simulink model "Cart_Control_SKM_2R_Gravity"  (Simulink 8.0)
settings: Solver=FixedStepDiscrete  SolverMode=SingleTasking  StartTime=0  StopTime=6  FixedStep=dt  RelTol=1e-3  SampleTimeConstraint=Specified
InitFcn:
  | % Sampling Times %
  | dt0=0.001; dt1=0.01; samples=10;
undefined symbols (not defined in the file or in its folder): DiscIntNeverNeededParam, Volts
libraries: simulink_extras x4, speedgoatlib_IO311 x3, speedgoatlib_IO101 x2, simulink x2, xpclib x1

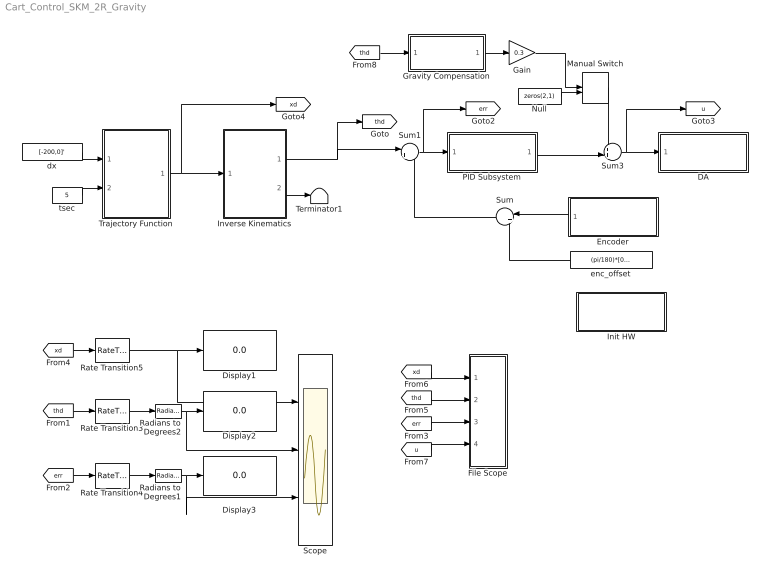
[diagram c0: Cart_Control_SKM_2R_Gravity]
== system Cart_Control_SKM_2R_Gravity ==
  DA : Subsystem  TreatAsAtomicUnit=on
  Display1 : Display
  Display2 : Display
  Display3 : Display
  Encoder : Subsystem  TreatAsAtomicUnit=on
  File Scope : Subsystem
  Gain : Gain  Gain=0.3
  Gravity Compensation : MATLAB Function  TreatAsAtomicUnit=on
  Init HW : Subsystem  TreatAsAtomicUnit=on
  Inverse Kinematics : MATLAB Function  TreatAsAtomicUnit=on
  Manual Switch : ManualSwitch
  Null : Constant  Value=zeros(2,1)
  PID Subsystem : Subsystem  TreatAsAtomicUnit=on
  Radians to Degrees1 : simulink_extras/Transformations/Radians to Degrees
  Radians to Degrees2 : simulink_extras/Transformations/Radians to Degrees
  Rate Transition3 : RateTransition  OutPortSampleTime=dt1
  Rate Transition4 : RateTransition  OutPortSampleTime=dt1
  Rate Transition5 : RateTransition  OutPortSampleTime=dt1
  Scope : Scope  NumInputPorts=3
  Sum : Sum  Inputs=|++
  Sum1 : Sum  Inputs=|+-
  Sum3 : Sum  Inputs=++|
  Terminator1 : Terminator
  Trajectory Function : MATLAB Function  TreatAsAtomicUnit=on
  dx : Constant  Value=[-200,0]'  SampleTime=dt0
  enc_offset : Constant  Value=(pi/180)*[0,90]'
  tsec : Constant  Value=5  SampleTime=dt0
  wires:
  Sum1/1 -> PID Subsystem/1(In1), [err]
  PID Subsystem/1(Out1) -> Sum3/2
  Encoder/1(Out1) -> Sum/1
  enc_offset/1 -> Sum/2
  Sum/1 -> Sum1/2
  [xd] -> File Scope/1(xd)
  [thd] -> File Scope/2(thd)
  [err] -> File Scope/3(err)
  [u] -> File Scope/4(u)
  dx/1 -> Trajectory Function/1(dx)
  tsec/1 -> Trajectory Function/2(tsec)
  Trajectory Function/1(xd) -> [xd], Inverse Kinematics/1(xd)
  Inverse Kinematics/1(thd) -> Sum1/1, [thd]
  [thd] -> Rate Transition3/1
  [err] -> Rate Transition4/1
  [xd] -> Rate Transition5/1
  Rate Transition5/1 -> Display1/1, Scope/1
  Rate Transition3/1 -> Radians to Degrees2/1
  Rate Transition4/1 -> Radians to Degrees1/1
  Radians to Degrees2/1 -> Display2/1, Scope/2
  Radians to Degrees1/1 -> Display3/1, Scope/3
  Inverse Kinematics/2(w_index) -> Terminator1/1
  Sum3/1 -> DA/1(In1), [u]
  Manual Switch/1 -> Sum3/1
  Null/1 -> Manual Switch/2
  [thd] -> Gravity Compensation/1(thd)
  Gravity Compensation/1(out) -> Gain/1
  Gain/1 -> Manual Switch/1

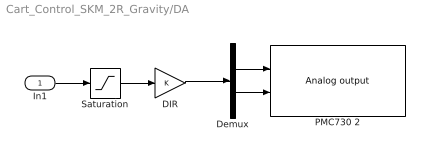
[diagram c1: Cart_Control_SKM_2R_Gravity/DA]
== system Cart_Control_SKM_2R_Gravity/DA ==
  In1 : Inport
  DIR : Gain
  Demux : Demux  Outputs=2
  PMC730 2 : speedgoatlib_IO101/Analog output  id=1  channel=[1,2]  reset=[1,1]  initValue=[0,0]  ts=dt0  pciSlot=-1
  Saturation : Saturate  UpperLimit=10  LowerLimit=-10
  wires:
  In1/1 -> Saturation/1
  Saturation/1 -> DIR/1
  DIR/1 -> Demux/1
  Demux/2 -> PMC730 2/2
  Demux/1 -> PMC730 2/1

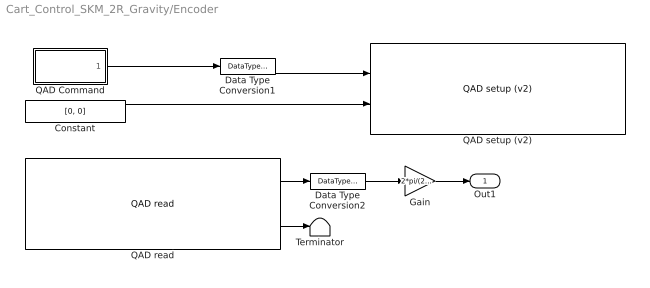
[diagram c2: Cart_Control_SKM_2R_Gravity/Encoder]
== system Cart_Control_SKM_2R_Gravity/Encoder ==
  Constant : Constant  Value=[0, 0]  OutDataTypeStr=Inherit: Inherit via back propagation
  Data Type Conversion1 : DataTypeConversion  OutDataTypeStr=uint8
  Data Type Conversion2 : DataTypeConversion  OutDataTypeStr=double
  Gain : Gain  Gain=2*pi/(23*2000)
  QAD Command : MATLAB Function  TreatAsAtomicUnit=on
  QAD read : speedgoatlib_IO311/QAD/QAD read  id=1  chan=[1 2]  pciSlot=-1  ts=dt0
  QAD setup (v2) : speedgoatlib_IO311/QAD/QAD setup (v2)  id=1  chan=[1,2]  debounce=0  quadrature=4x  index=Ignore index input  special=Disabled (cycling counter)  steps=2000  ts=dt0  pciSlot=-1
  Terminator : Terminator
  Out1 : Outport
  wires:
  Gain/1 -> Out1/1
  Constant/1 -> QAD setup (v2)/2
  QAD read/2 -> Terminator/1
  QAD read/1 -> Data Type Conversion2/1
  QAD Command/1(y) -> Data Type Conversion1/1
  Data Type Conversion2/1 -> Gain/1
  Data Type Conversion1/1 -> QAD setup (v2)/1

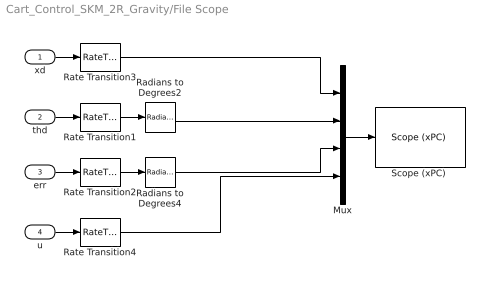
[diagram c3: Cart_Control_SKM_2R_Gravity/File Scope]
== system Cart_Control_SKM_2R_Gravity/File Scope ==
  xd : Inport
  thd : Inport  Port=2
  err : Inport  Port=3
  u : Inport  Port=4
  Mux : Mux
  Radians to Degrees2 : simulink_extras/Transformations/Radians to Degrees
  Radians to Degrees4 : simulink_extras/Transformations/Radians to Degrees
  Rate Transition{1..4} (4 alike) : RateTransition  OutPortSampleTime=dt1
  "Scope (xPC) " : xpclib/Misc./Scope (xPC)   scopeno=1  scopetype=File  autostart=on  viewmode=Graphical redraw  formatstr='%15.6f'  grid=on  ylimits=[0,0]  nosamples=100  noprepostsamples=0  interleave=1  triggermode=FreeRun  triggersignal=1  triggerlevel=0.0  triggerslope=Either  triggerscope=1  triggersample=0  filename=step2.dat  mode=Lazy  writesize=512  autorestart=on  dynamicfilemode=off  maxwritefilesize=512*1024^2
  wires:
  Radians to Degrees2/1 -> Mux/2
  Radians to Degrees4/1 -> Mux/3
  Rate Transition1/1 -> Radians to Degrees2/1
  Rate Transition2/1 -> Radians to Degrees4/1
  thd/1 -> Rate Transition1/1
  err/1 -> Rate Transition2/1
  Rate Transition3/1 -> Mux/1
  xd/1 -> Rate Transition3/1
  u/1 -> Rate Transition4/1
  Mux/1 -> "Scope (xPC) "/1
  Rate Transition4/1 -> Mux/4

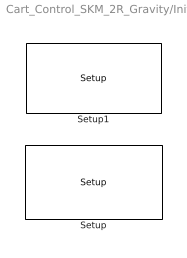
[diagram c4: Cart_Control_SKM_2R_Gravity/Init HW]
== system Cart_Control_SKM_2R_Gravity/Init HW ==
  Setup : speedgoatlib_IO311/Setup/Setup  group=Module setup  id=1  fpga1=speedgoat_IO311_default  pciSlot=-1  lowerDirection=[1 1 1 1 1 0 0 0 0 0 0 0 1 0 0 0]  lowerReset=[1]  lowerValue=[0]  upperDirection=[1 1 1 1 1 1 1 1 1 0 0 0 0 0 0 0]  upperReset=[1]  upperValue=[0]
  Setup1 : speedgoatlib_IO101/Setup  group=Module setup  id=1  pciSlot=-1  adStartChannel=1  adNumChannel=32  adCoupling=Single-ended  adRange=-10 .. 10 Volts  adAcqMode=Standard  daChannel=[1,2]  daReset=[1,1]  daInitValue=[0,0]  lowerChannel=1  lowerDirection=Input  lowerDIDebounce=0  lowerDOReset=[1]  lowerDOInitValues=[0]  upperChannel=1  upperDirection=Output  upperDIDebounce=0  upperDOReset=0  upperDOInitValues=0

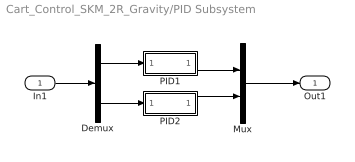
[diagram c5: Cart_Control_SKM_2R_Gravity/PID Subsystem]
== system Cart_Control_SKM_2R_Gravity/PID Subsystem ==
  In1 : Inport
  Demux : Demux  Outputs=2
  Mux : Mux  Inputs=2
  PID1 : Subsystem
  PID2 : Subsystem
  Out1 : Outport
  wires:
  In1/1 -> Demux/1
  Demux/1 -> PID1/1(In1)
  PID1/1(Out1) -> Mux/1
  Demux/2 -> PID2/1(In1)
  PID2/1(Out1) -> Mux/2
  Mux/1 -> Out1/1

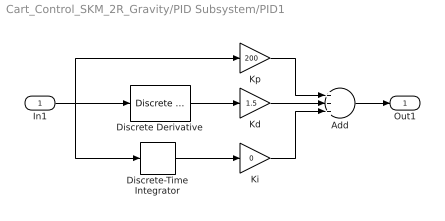
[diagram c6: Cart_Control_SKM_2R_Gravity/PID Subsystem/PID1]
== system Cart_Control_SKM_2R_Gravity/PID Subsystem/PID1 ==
  In1 : Inport
  Add : Sum  Inputs=+++
  Discrete Derivative : simulink/Discrete/Discrete Derivative  gainval=1.0  ICPrevScaledInput=0.0  InputProcessing=Inherited  OutMin=[]  OutMax=[]  OutDataType=fixdt(1, 16)  OutScaling=2^-10  DoSatur=off
  Discrete-Time Integrator : DiscreteIntegrator  SampleTime=dt0  ICPrevOutput=DiscIntNeverNeededParam  ICPrevScaledInput=DiscIntNeverNeededParam
  Kd : Gain  Gain=1.5
  Ki : Gain  Gain=0
  Kp : Gain  Gain=200
  Out1 : Outport
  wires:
  Discrete-Time Integrator/1 -> Ki/1
  Kp/1 -> Add/1
  Kd/1 -> Add/2
  Ki/1 -> Add/3
  Discrete Derivative/1 -> Kd/1
  Add/1 -> Out1/1
  In1/1 -> Kp/1, Discrete Derivative/1, Discrete-Time Integrator/1

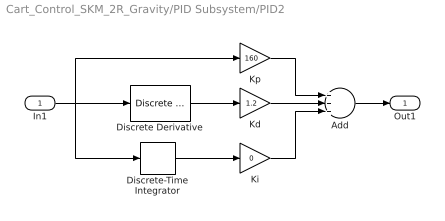
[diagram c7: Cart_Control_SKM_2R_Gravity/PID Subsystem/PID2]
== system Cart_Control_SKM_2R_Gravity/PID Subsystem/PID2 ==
  In1 : Inport
  Add : Sum  Inputs=+++
  Discrete Derivative : simulink/Discrete/Discrete Derivative  gainval=1.0  ICPrevScaledInput=0.0  InputProcessing=Inherited  OutMin=[]  OutMax=[]  OutDataType=fixdt(1, 16)  OutScaling=2^-10  DoSatur=off
  Discrete-Time Integrator : DiscreteIntegrator  SampleTime=dt0  ICPrevOutput=DiscIntNeverNeededParam  ICPrevScaledInput=DiscIntNeverNeededParam
  Kd : Gain  Gain=1.2
  Ki : Gain  Gain=0
  Kp : Gain  Gain=160
  Out1 : Outport
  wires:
  Discrete-Time Integrator/1 -> Ki/1
  Kp/1 -> Add/1
  Kd/1 -> Add/2
  Ki/1 -> Add/3
  Discrete Derivative/1 -> Kd/1
  Add/1 -> Out1/1
  In1/1 -> Kp/1, Discrete Derivative/1, Discrete-Time Integrator/1

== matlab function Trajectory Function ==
function xd = fcn(dx, tsec)

persistent index xd_p

MAX_CH=2;       % Two Actuators %
dt=0.001;       % Step time is 10 msec %
a1=100; a2=100;

% Initializing Variables %
if isempty(index), index=0; end
if isempty(xd_p), xd_p=zeros(MAX_CH,1); end
xd=zeros(MAX_CH,1);
x0=[a1,a2]';

tout=index*dt;
if index<(tsec/dt)
    [c] = coeff_3rd(x0, zeros(MAX_CH,1), x0+dx, zeros(MAX_CH,1), tsec);
    for ch=1:MAX_CH
        xd(ch,1)=c(ch,1)+c(ch,2)*tout+c(ch,3)*tout^2+c(ch,4)*tout^3;    
    end
    xd_p=xd;
else
    xd=xd_p;
end
index=index+1;

function [c] = coeff_3rd(sp, sv, ep, ev, tsec)
MAX_CH=2;
c=zeros(MAX_CH,4);
for ch=1:MAX_CH
    c(ch,1)=sp(ch,1);
    c(ch,2)=sv(ch,1);
    c(ch,3)=(3.0*(ep(ch,1)-sp(ch,1))-(2.0*sv(ch,1)+ev(ch,1))*tsec)/(tsec*tsec);
    c(ch,4)=(-2.0*(ep(ch,1)-sp(ch,1))+(sv(ch,1)+ev(ch,1))*tsec)/(tsec*tsec*tsec);
end

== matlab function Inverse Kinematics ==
function [thd,w_index]  = fcn(xd)

persistent index thd_p

% Initializing Variables %
if isempty(index), index=0; end
if isempty(thd_p), thd_p=(pi/180)*[0,90]'; end

w_index=1;  % In workspace %
a1=100; a2=100;

% (1) Calculate th2 %
px=xd(1,1); py=xd(2,1);
kapha=(px^2+py^2-a1^2-a2^2)/(2*a1*a2);
if abs(kapha)>1
    w_index=-1;  % Out of Workspace %
    kapha=1;
end
th2=+acos(kapha); % Elbow Down %
%th2=-acos(kapha); % Elbow Up %
 
% (2) Calculate th1 %
delta=a1^2+a2^2+2*a1*a2*cos(th2);
cth1=(px*(a1+a2*cos(th2))+py*a2*sin(th2))/delta;
sth1=(-px*a2*sin(th2)+py*(a1+a2*cos(th2)))/delta;
th1=atan2(sth1, cth1);
if th1<0, th1=th1+2*pi; end % 0<th<360 %

% (3) Check Joint Limits %
if th1<0 || th1>pi, w_index=-1; end
if th2<pi/6 || th2>5*pi/6, w_index=-1; end

% Result %
if w_index==1
    thd=[th1, th2]';
else
    thd=thd_p;
end

% Save the current value %
thd_p=thd;

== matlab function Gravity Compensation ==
function out = fcn(thd)

MM2M=0.001;

th1=thd(1,1); th2=thd(2,1);
tau=zeros(2,1); out=zeros(2,1);

m1=0.363; a1=MM2M*100; ac1=MM2M*87.74;
m2=0.075; ac2=MM2M*41.68;
g=-9.81;    % Gravity Direction -Y axis %

tau(1,1)=g*(m1*ac1*cos(th1)+m2*(a1*cos(th1)+ac2*cos(th1+th2)));
tau(2,1)=m2*g*ac2*cos(th1+th2);

% Motor Torque Gain 10[V]/Max Torque[Nm] %
ratio=66/23;

out(1,1)=tau(1,1);
out(2,1)=ratio*tau(2,1);

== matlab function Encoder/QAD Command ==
function y = fcn()

persistent index

if isempty(index), index=0; end

if index==0
    y=[1,1];      %  Reset %
else
    y = [0,0];
end

index=index+1;
